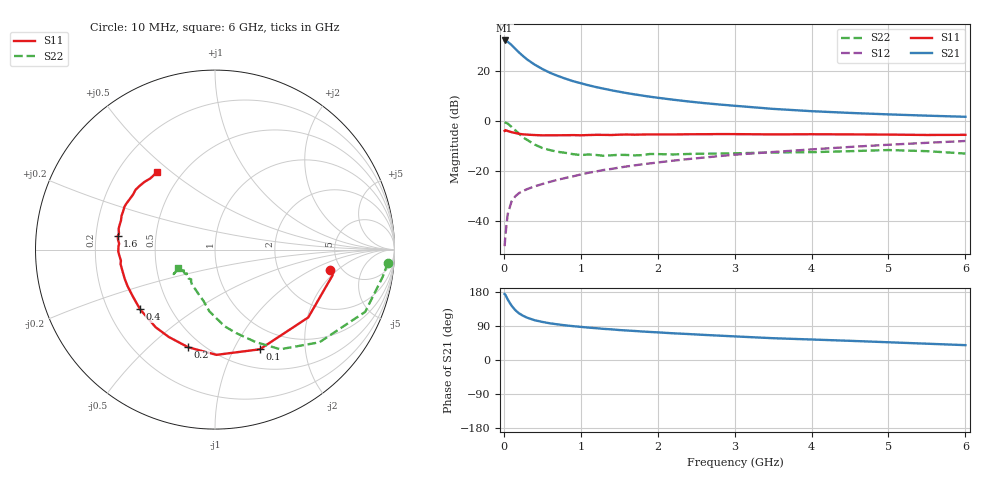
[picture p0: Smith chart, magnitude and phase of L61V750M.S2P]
!  INFINEON TECHNOLOGIES Small Signal Semiconductors
! BFR380L3 , Si-NPN RF-Transistor in TSLP-3-1
!  Vce=1.75 V,  Ic=50 mA
! Common Emitter S-Parameters:  07. March 2005
#  GHz  S  MA  R  50
! f  S11  S21  S12  S22
! GHz  Mag  Ang  Mag  Ang  Mag  Ang  Mag  Ang
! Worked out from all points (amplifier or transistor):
!   36 points, 10 MHz to 6 GHz, reference 50 ohm
!   highest |S21| = 32.4 dB at 10 MHz (marker M1)
!   |S21| within 3 dB of that: start of sweep to 138.3 MHz
!   unconditionally stable (mu >= 1): 1.556 GHz to 4.946 GHz
!   at 250 MHz: K = 0.47, MSG = 27.0 dB, |S12| = -27.8 dB
!   at 1.4 GHz: K = 0.99, MSG = 15.7 dB, |S12| = -19.0 dB
!   at 6 GHz: K = 0.98, MSG = 4.8 dB, |S12| = -7.8 dB
!   S11 on the Smith chart (normalised r, x): 10 MHz: 4.05, -1.56; 100 MHz: 0.72, -1.27; 200 MHz: 0.42, -0.67; 400 MHz: 0.34, -0.31; 1.6 GHz: 0.29, +0.06; 6 GHz: 0.37, +0.44
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0.01  0.6481 -9.9  41.58 174.1  0.0032 69.9  0.966 -4.3
0.02  0.671 -12.2  41.28 172.0  0.0052 85.0  0.9464 -9.2
0.05  0.6425 -36.0  39.15 159.8  0.014 76.4  0.906 -22.5
0.1  0.609 -65.8  33.73 143.4  0.0251 63.2  0.7779 -41.6
0.15  0.5865 -89.2  28.24 131.3  0.032 57.6  0.6635 -56.8
0.2  0.5643 -105.3  23.69 122.8  0.0371 54.7  0.5624 -66.3
0.25  0.5507 -117.9  20.25 116.7  0.0406 51.9  0.4789 -75.9
0.3  0.5445 -127.4  17.46 111.9  0.0441 52.0  0.4302 -82.9
0.4  0.5339 -141.4  13.69 105.0  0.0503 52.3  0.3451 -95.3
0.5  0.5269 -150.6  11.2 100.5  0.0559 54.5  0.2941 -102.4
0.6  0.5279 -157.3  9.389 96.8  0.062 56.1  0.2669 -109.5
0.7  0.5287 -162.1  8.14 94.0  0.0681 58.0  0.2465 -116.4
0.9  0.5323 -171.2  6.38 89.3  0.0797 60.3  0.2214 -127.2
1.1  0.534 -176.4  5.282 85.5  0.0938 62.7  0.2182 -132.5
1.3  0.538 178.1  4.506 82.1  0.1071 63.2  0.2052 -140.0
1.6  0.5475 172.1  3.68 77.8  0.1259 64.2  0.2133 -146.2
2.2  0.5482 163.0  2.718 70.5  0.1641 64.9  0.2184 -148.0
2.8  0.5581 154.6  2.18 64.3  0.2022 64.9  0.2275 -152.9
3.5  0.5499 146.3  1.781 57.5  0.2446 62.7  0.239 -151.4
4.5  0.5502 140.1  1.479 50.6  0.3087 60.8  0.254 -150.4
5.5  0.5357 132.1  1.303 43.0  0.3733 56.7  0.2541 -150.3
6  0.5389 127.0  1.238 39.2  0.406 54.4  0.2277 -153.6
